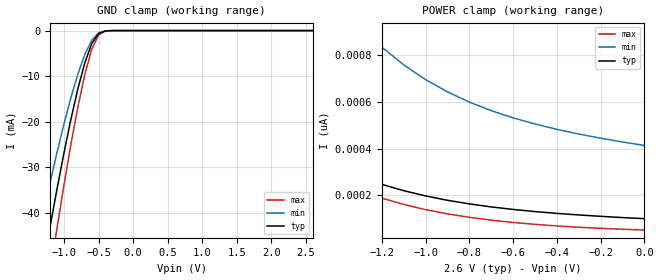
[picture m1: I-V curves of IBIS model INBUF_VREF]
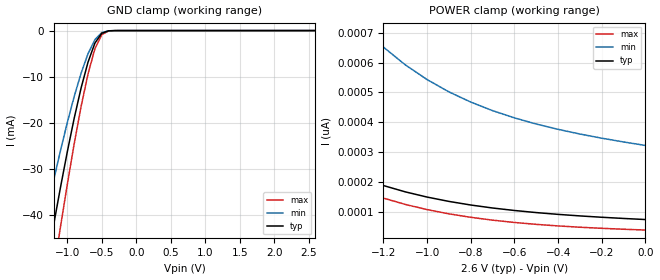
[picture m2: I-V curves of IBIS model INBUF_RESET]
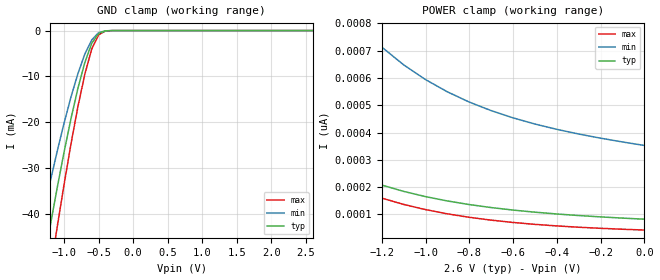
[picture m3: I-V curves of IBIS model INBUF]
| IBIS file sstvn859_mlf_3200.ibs created by s2ibis2 version 1.2
| North Carolina State University Electronics Research Laboratory  1995
[IBIS ver]   2.1
[File name]   sstvn859_mlf_3200.ibs
[File Rev]   1.0
[Date]   Thursday, November 6, 2003
[Source]   IDT
[Notes]   1. Temp typ=25C, min=0C, max=70C
   2. IDT's 2.0v C11.5 process
   3. Ramp rate based on 50 ohm load
READ THESE TERMS AND CONDITIONS CAREFULLY BEFORE USING THIS IBIS MODEL.  BY
USING THIS IBIS MODEL, YOU ARE ACCEPTING AND AGREEING TO THESE TERMS AND
CONDITIONS OF USE.
Integrated Device Technology, Inc. ("IDT") hereby grants the user of this
IBIS model ("User") a non-exclusive, nontransferable license to use this
IBIS model under the following terms: The User is granted this license only
to use the IBIS model for demonstration purposes only and is not granted
rights to sell, copy (except as needed to run the IBIS model), rent, lease
or sub-license (except for demonstration) the IBIS model in whole or in
part, or in modified form to anyone. The User may modify the IBIS model to
suit its specific applications, but  rights to derivative works and such
modifications shall belong to IDT.
THIS IBIS MODEL IS PROVIDED ON AN AS IS" BASIS AND IDT  MAKES ABSOLUTELY NO
WARRANTY WITH RESPECT TO THE INFORMATION CONTAINED HEREIN.  IDT DISCLAIMS
AND USER WAIVES ALL WARRANTIES, EXPRESS AND IMPLIED, INCLUDING WARRANTIES OF
MERCHANTABILITY AND FITNESS FOR A PARTICULAR PURPOSE.  THE ENTIRE RISK AS TO
QUALITY AND PERFORMANCE IS WITH THE USER  ACCORDINGLY, IN NO EVENT SHALL IDT
BE LIABLE FOR ANY DIRECT OR INDIRECT DAMAGES, WHETHER IN CONTRACT OR TORT,
INCLUDING ANY LOST PROFITS OR OTHER INCIDENTAL, CONSEQUENTIAL, EXEMPLARY, OR
PUNITIVE DAMAGES ARISING OUT OF THE USE OR APPLICATION OF THE  IBIS MODEL,
WHETHER OR NOT IDT HAD NOTICE OF SUCH DAMAGES.
IDT reserves the right to make changes without notice to any product herein
to improve reliability, function, or design. IDT does not convey any license
under patent rights or any other intellectual property rights, including
those of third parties. IDT is not obligated to provide maintenance or
support for the licensed IBIS model.
This model is for the 13-Bit to 26-Bit Registered Buffer With SSTL I/O
configuration
[Copyright]
Copyright 2002, Integrated Device Technology, Inc. All rights reserved.
|   Component IDT74SSTVN16859
[Component]   IDT74SSTVN16859
[Manufacturer]   Integrated Device Technology Inc.
[Package]
|Following package parameters are for 56 lead MLF package
| variable   typ   min   max
R_pkg   0.11300   87.30000m   0.15140
L_pkg   2.59000nH   1.99000nH   3.46400nH
C_pkg   0.19900pF   0.15600pF   0.25600pF
[Pin]  signal_name   model_name   R_pin   L_pin   C_pin
1   Q7A   OUTBUF
2   Q6A   OUTBUF
3   Q5A   OUTBUF
4   Q4A   OUTBUF
5   Q3A   OUTBUF
6   Q2A   OUTBUF
7   Q1A   OUTBUF
8   Q13B   OUTBUF
9   VDDQ   POWER
10   Q12B   OUTBUF
11   Q11B   OUTBUF
12   Q10B   OUTBUF
13   Q9B   OUTBUF
14   Q8B   OUTBUF
15   Q7B   OUTBUF
16   Q6B   OUTBUF
17   VDDQ   POWER
18   Q5B   OUTBUF
19   Q4B   OUTBUF
20   Q3B   OUTBUF
21   Q2B   OUTBUF
22   Q1B   OUTBUF
23   VDDQ   POWER
24   D1   INBUF
25   D2   INBUF
26   VDD   POWER
27   VDDQ   POWER
28   D3   INBUF
29   D4   INBUF
30   D5   INBUF
31   D6   INBUF
32   VREF   INBUF_VREF
33   VDD   POWER
34   VDDQ   POWER
35   CLK   INBUF_CLK
36   _CLK_   INBUF_CLK
37   GND   GND
38   _RESET_   INBUF_RESET
39   D7   INBUF
40   D8   INBUF
41   D9   INBUF
42   D10   INBUF
43   D11   INBUF
44   VDDQ   POWER
45   VDD   POWER
46   D12   INBUF
47   D13   INBUF
48   GND   INBUF
49   VDDQ   POWER
50   Q13A   OUTBUF
51   Q12A   OUTBUF
52   Q11A   OUTBUF
53   Q10A   OUTBUF
54   Q9A   OUTBUF
55   VDDQ   POWER
56   Q8A   OUTBUF
| in   in   dummy_model
[Diff Pin]  inv_pin  vdiff   tdelay_typ  tdelay_min  tdelay_max
35   36   0.36000V  NA | CLK/CLKB pins
[Pin Mapping]  pulldown_ref   pullup_ref   gnd_clamp_ref  power_clamp_ref
1   GND   VDDQ
2   GND   VDDQ
3   GND   VDDQ
4   GND   VDDQ
5   GND   VDDQ
6   GND   VDDQ
7   GND   VDDQ
8   GND   VDDQ
9   NC   VDDQ
10   GND   VDDQ
11   GND   VDDQ
12   GND   VDDQ
13   GND   VDDQ
14   GND   VDDQ
15   GND   VDDQ
16   GND   VDDQ
17   NC   VDDQ
18   GND   VDDQ
19   GND   VDDQ
20   GND   VDDQ
21   GND   VDDQ
22   GND   VDDQ
23   NC   VDDQ
24   NC   NC   GND   VDDQ
25   NC   NC   GND   VDDQ
26   NC   VDD
27   NC   VDDQ
28   NC   NC   GND   VDDQ
29   NC   NC   GND   VDDQ
30   NC   NC   GND   VDDQ
31   NC   NC   GND   VDDQ
32   NC   NC   GND   VDDQ
33   NC   VDD
34   NC   VDDQ
35   NC   NC   GND   VDDQ
36   NC   NC   GND   VDDQ
37   GND   NC
38   NC   NC   GND   VDDQ
39   NC   NC   GND   VDDQ
40   NC   NC   GND   VDDQ
41   NC   NC   GND   VDDQ
42   NC   NC   GND   VDDQ
43   NC   NC   GND   VDDQ
44   NC   VDDQ
45   NC   VDD
46   NC   NC   GND   VDDQ
47   NC   NC   GND   VDDQ
48   GND   NC
49   NC   VDDQ
50   GND   VDDQ
51   GND   VDDQ
52   GND   VDDQ
53   GND   VDDQ
54   GND   VDDQ
55   NC   VDDQ
56   GND   VDDQ
| Models and submodels in the file (5): INBUF_VREF (Input), INBUF_RESET (Input), INBUF (Input), INBUF_CLK (Input), OUTBUF (Output)
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|   Model INBUF_VREF
[Model]   INBUF_VREF
Model_type   Input
Polarity   Non-Inverting
Vinl =  1.25000V
Vinh =  1.35000V
C_comp   2.50000pF   2.50000pF   2.50000pF
[Temperature Range]   25.00000   70.00000   0.000
[Voltage Range]   2.60000V   2.50000V   2.70000V
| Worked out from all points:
|   GND clamp passes 1 mA (typ) near -0.52 V on its own axis
[GND_clamp]
| voltage   I(typ)   I(min)   I(max)
-2.6V     -168.7mA   -138.9mA   -194.7mA
-1.4V     -60.05mA   -47.14mA   -72.86mA
-1.3V     -51.32mA   -40.05mA   -62.76mA
-1.2V     -42.8mA    -33.18mA   -52.81mA
-1.1V     -34.56mA   -26.6mA    -43.11mA
-900mV    -19.37mA   -14.66mA   -24.89mA
-800mV    -12.74mA   -9.544mA   -16.75mA
-700mV    -7.091mA   -5.252mA   -9.645mA
-600mV    -2.871mA   -2.118mA   -4.115mA
-500mV    -637.8uA   -495.3uA   -959.3uA
-300mV    -3.063uA   -4.006uA   -3.923uA
2.6V      98.9pA     428.4pA    47.06pA
[POWER_clamp]
| voltage   I(typ)   I(min)   I(max)
-2.6V     1.876nA    5.37nA     1.896nA
-2.2V     1.035nA    3.042nA    1.003nA
-2.1V     889.8pA    2.636nA    850.6pA
-2V       764.4pA    2.286nA    719.6pA
-1.9V     656.9pA    1.985nA    607.8pA
-1.7V     487pA      1.509nA    432.1pA
-1.5V     365.1pA    1.168nA    307.2pA
-1.3V     279.1pA    927.1pA    219.9pA
-1V       196.6pA    696.1pA    137.8pA
-800mV    162.4pA    599.6pA    104.7pA
-500mV    129.4pA    505.4pA    74.47pA
0V        98.9pA     413.4pA    50.09pA
|   Model INBUF_RESET
[Model]   INBUF_RESET
Model_type   Input
Polarity   Non-Inverting
Vinl =  0.70000V
Vinh =  1.70000V
C_comp   2.50000pF   2.50000pF   2.50000pF
[Temperature Range]   25.00000   70.00000   0.000
[Voltage Range]   2.60000V   2.50000V   2.70000V
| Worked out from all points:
|   GND clamp passes 1 mA (typ) near -0.52 V on its own axis
[GND_clamp]
| voltage   I(typ)   I(min)   I(max)
-2.6V     -167.2mA   -137.2mA   -193.3mA
-1.4V     -59.32mA   -46.36mA   -72.17mA
-1.3V     -50.66mA   -39.34mA   -62.13mA
-1.2V     -42.21mA   -32.55mA   -52.25mA
-1.1V     -34.04mA   -26.05mA   -42.6mA
-900mV    -18.98mA   -14.27mA   -24.51mA
-800mV    -12.43mA   -9.231mA   -16.44mA
-700mV    -6.859mA   -5.022mA   -9.408mA
-600mV    -2.718mA   -1.972mA   -3.951mA
-500mV    -567.1uA   -431.8uA   -874.7uA
-300mV    -2.396uA   -3.132uA   -3.069uA
2.6V      74.28pA    334.2pA    36.7pA
[POWER_clamp]
| voltage   I(typ)   I(min)   I(max)
-2.6V     1.459nA    4.19nA     1.48nA
-2.2V     802.9pA    2.373nA    783.1pA
-2.1V     689.4pA    2.056nA    663.8pA
-2V       591.6pA    1.783nA    561.6pA
-1.9V     507.7pA    1.549nA    474.3pA
-1.7V     375.3pA    1.178nA    337.2pA
-1.5V     280.4pA    911.3pA    239.7pA
-1.3V     213.5pA    723.3pA    171.6pA
-1V       149.5pA    543.1pA    107.5pA
-800mV    122.9pA    467.8pA    81.69pA
-500mV    97.55pA    394.3pA    58.09pA
0V        74.28pA    322.6pA    39.06pA
|   Model INBUF
[Model]   INBUF
Model_type   Input
Polarity   Non-Inverting
Vinl =  0.94000V
Vinh =  1.66000V
C_comp   2.50000pF   2.50000pF   2.50000pF
[Temperature Range]   25.00000   70.00000   0.000
[Voltage Range]   2.60000V   2.50000V   2.70000V
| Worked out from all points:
|   GND clamp passes 1 mA (typ) near -0.52 V on its own axis
[GND_clamp]
| voltage   I(typ)   I(min)   I(max)
-2.6V     -168.1mA   -138.2mA   -194.1mA
-1.4V     -59.73mA   -46.79mA   -72.56mA
-1.3V     -51.03mA   -39.73mA   -62.48mA
-1.2V     -42.53mA   -32.89mA   -52.56mA
-1.1V     -34.32mA   -26.35mA   -42.88mA
-900mV    -19.19mA   -14.47mA   -24.71mA
-800mV    -12.59mA   -9.39mA    -16.6mA
-700mV    -6.975mA   -5.134mA   -9.529mA
-600mV    -2.79mA    -2.039mA   -4.03mA
-500mV    -596.8uA   -457.6uA   -911.7uA
-300mV    -2.619uA   -3.425uA   -3.355uA
2.6V      82.49pA    365.6pA    40.15pA
[POWER_clamp]
| voltage   I(typ)   I(min)   I(max)
-2.6V     1.598nA    4.583nA    1.618nA
-2.2V     880.4pA    2.596nA    856.5pA
-2.1V     756.2pA    2.249nA    726.1pA
-2V       649.2pA    1.951nA    614.3pA
-1.9V     557.4pA    1.694nA    518.8pA
-1.7V     412.5pA    1.288nA    368.8pA
-1.5V     308.6pA    996.8pA    262.2pA
-1.3V     235.3pA    791.2pA    187.7pA
-1V       165.2pA    594.1pA    117.6pA
-800mV    136.1pA    511.7pA    89.36pA
-500mV    108.2pA    431.3pA    63.55pA
0V        82.49pA    352.8pA    42.73pA
